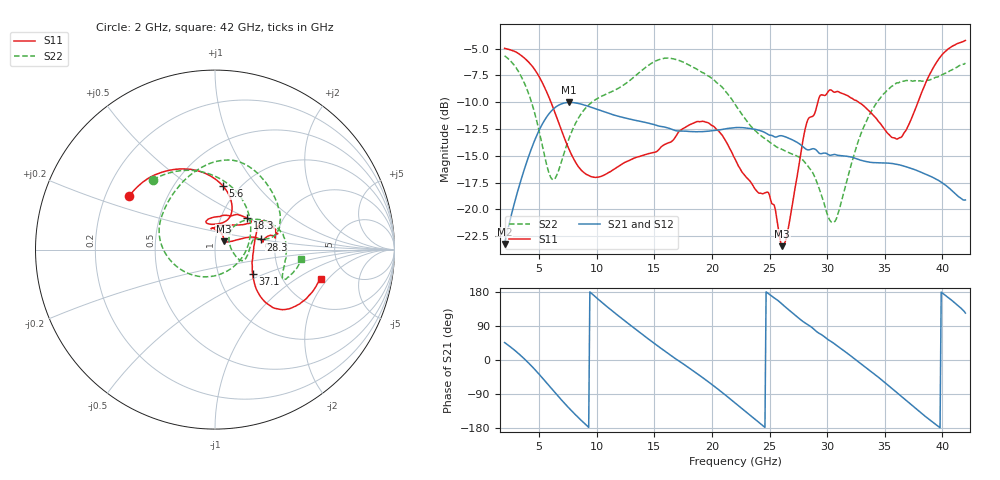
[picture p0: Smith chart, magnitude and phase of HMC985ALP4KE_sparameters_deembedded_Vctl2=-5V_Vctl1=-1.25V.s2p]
!s2p File: Measurements: S11, S21, S12, S22
# GHz S dB R 50.0
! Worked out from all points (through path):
!   401 points, 2 GHz to 42 GHz, reference 50 ohm
!   highest |S21| = -10.02 dB at 7.6 GHz (marker M1); lowest = -23.2 dB at 2 GHz (marker M2)
!   lowest |S11| = -23.4 dB at 26.1 GHz (marker M3), VSWR 1.14, Z = 54.9 + j5.05 ohm
!   |S11| at or under -10 dB: 6.024 GHz to 29.18 GHz (23.16 GHz wide, 132 % of centre); 32.72 GHz to 37.88 GHz (5.162 GHz wide, 14.6 % of centre)
!   |S22| runs from -21.2 to -5.7 dB; largest |S21 - S12| = 0.00032
!   S11 on the Smith chart (normalised r, x): 2 GHz: 0.30, +0.26; 5.6 GHz: 0.84, +0.68; 18.3 GHz: 1.33, +0.50; 28.3 GHz: 1.66, +0.20; 37.1 GHz: 1.46, -0.42; 42 GHz: 3.21, -1.70
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2  -4.98 148.0  -23.24 46.0  -23.25 46.0  -5.67 131.7
3.6  -5.78 121.4  -16.65 6.2  -16.65 6.2  -7.95 87.3
4.7  -7.10 100.5  -13.34 -27.6  -13.34 -27.6  -11.38 45.4
5.6  -8.92 83.0  -11.46 -58.6  -11.47 -58.6  -15.62 -7.9
6.4  -11.06 70.9  -10.48 -86.9  -10.49 -86.9  -17.09 -76.8
7.6  -14.42 66.1  -10.02 -127.3  -10.03 -127.3  -13.36 -146.8
8.7  -16.40 76.5  -10.20 -160.7  -10.20 -160.7  -11.00 -177.6
12  -15.91 108.2  -11.35 113.6  -11.36 113.7  -8.63 135.8
15.4  -14.41 79.9  -12.23 34.7  -12.24 34.7  -6.03 85.1
18.3  -12.00 44.3  -12.75 -27.1  -12.76 -27.1  -6.70 50.3
20.3  -12.43 37.7  -12.62 -71.8  -12.63 -71.8  -8.05 23.6
22  -15.29 52.9  -12.38 -113.3  -12.38 -113.3  -10.18 11.8
24.9  -18.43 95.3  -13.03 175.1  -13.04 175.2  -13.64 10.7
26.1  -23.44 42.9  -13.14 147.2  -13.15 147.2  -14.42 -2.1
28.3  -11.70 12.5  -14.45 93.7  -14.45 93.7  -15.93 -22.6
28.7  -11.34 9.1  -14.36 85.3  -14.36 85.3  -16.48 -22.6
30.6  -9.07 15.7  -14.88 43.3  -14.88 43.4  -21.19 21.3
33.1  -10.28 31.3  -15.47 -13.7  -15.48 -13.6  -12.49 43.9
35.4  -13.05 8.9  -15.70 -69.4  -15.70 -69.3  -8.72 19.5
37.1  -12.06 -32.9  -16.12 -113.0  -16.12 -113.0  -8.00 0.0
39.7  -5.95 -41.6  -17.32 -176.5  -17.32 -176.4  -7.58 -23.6
42  -4.24 -15.6  -19.13 123.8  -19.13 123.9  -6.34 -6.0
